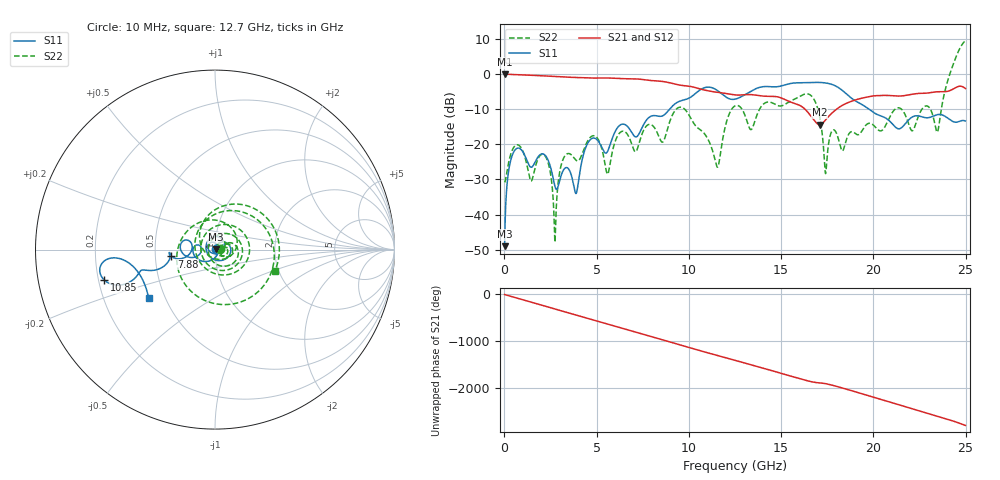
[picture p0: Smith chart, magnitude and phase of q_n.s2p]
!Keysight Technologies,N5245B,MY57181346,A.12.70.07
!Automatic Fixture Removal (AFR)
!Date: Wednesday, November 07, 2018 11:51:34 AM
!S2P File: Measurements: S11,S21,S12,S22:
# MHz S  RI  R 50
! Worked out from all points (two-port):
!   2499 points, 10 MHz to 24.99 GHz, reference 50 ohm
!   highest |S21| = 0.00 dB at 10 MHz (marker M1); lowest = -14.4 dB at 17.09 GHz (marker M2)
!   |S21| within 3 dB of the highest: start of sweep to 9.377 GHz
!   lowest |S11| = -49.0 dB at 10 MHz (marker M3), VSWR 1.01, Z = 50.3 + j0.187 ohm
!   |S11| at or under -10 dB: start of sweep to 8.952 GHz; 19.76 GHz to end of sweep
!   |S22| runs from -47.9 to 9.6 dB; largest |S21 - S12| = 1.4e-15
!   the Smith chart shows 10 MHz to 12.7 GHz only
!   S11 on the Smith chart (normalised r, x): 10 MHz: 1.01, +0.00; 7.88 GHz: 0.61, -0.05; 10.85 GHz: 0.22, -0.13; 12.7 GHz: 0.41, -0.28
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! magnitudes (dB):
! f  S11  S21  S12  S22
! 10 MHz  -49.0  0.0  0.0  -30.8
! 240 MHz  -27.2  -0.1  -0.1  -24.9
! 630 MHz  -21.3  -0.2  -0.2  -20.2
! 1.44 GHz  -26.5  -0.3  -0.3  -30.5
! 2.24 GHz  -23.3  -0.5  -0.5  -23.6
! 2.74 GHz  -32.0  -0.7  -0.7  -47.9
! 3.2 GHz  -27.3  -0.8  -0.8  -24.0
! 4.18 GHz  -25.2  -1.0  -1.0  -23.2
! 5.6 GHz  -21.9  -1.1  -1.1  -28.5
! 7.88 GHz  -12.2  -1.8  -1.8  -14.3
! 8.34 GHz  -12.0  -2.0  -2.0  -17.4
! 9.54 GHz  -7.6  -3.2  -3.2  -9.4
! 10.85 GHz  -3.9  -4.5  -4.5  -17.0
! 11.56 GHz  -4.7  -5.2  -5.2  -26.5
! 12.5 GHz  -7.1  -5.9  -5.9  -9.0
! 12.7 GHz  -6.8  -6.0  -6.0  -9.0
! 16.67 GHz  -2.4  -12.3  -12.3  -6.4
! 17.09 GHz  -2.4  -14.4  -14.4  -12.1
! 17.42 GHz  -2.5  -13.0  -13.0  -28.2
! 20.83 GHz  -13.1  -6.1  -6.1  -12.8
! 23.47 GHz  -11.5  -5.0  -5.0  -16.5
! 24.99 GHz  -13.4  -4.1  -4.1  9.6
